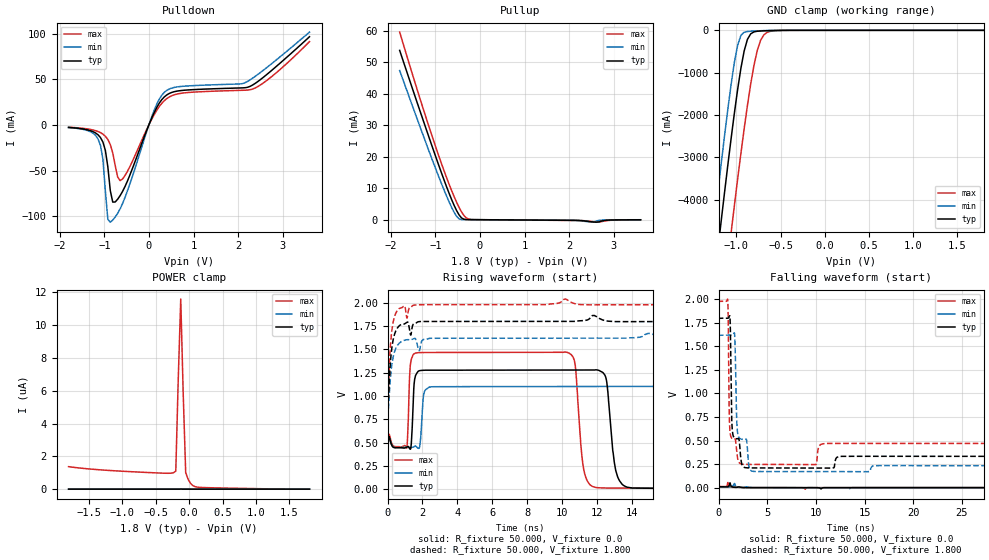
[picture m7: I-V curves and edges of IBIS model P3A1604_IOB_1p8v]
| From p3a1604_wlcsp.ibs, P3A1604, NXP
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[Model] P3A1604_IOB_1p8v
Model_type I/O
Polarity   Non-Inverting
Enable   Active-High
Vinl =  0.7915V
Vinh =  0.9305V
C_comp   5.4pF   5pF   5.9pF
[Model Spec]
Vinh   0.9305V   0.7875V   1.094V
Vinl   0.7915V   0.6765V   0.8965V
[Temperature Range]   27.000   -40.000   125
[Voltage Range]   1.800V   1.620V   1.980V
[Pullup Reference]   1.800V   1.620V   1.980V
[Pulldown Reference]   0.0V   0.0V   0.0V
[POWER Clamp Reference]   1.800V   1.620V   1.980V
[GND Clamp Reference]   0.0V   0.0V   0.0V
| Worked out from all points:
|   slope of the pulldown table from 0 to 0.27 V, typ, clamps not added: 10.2 ohm
|   slope of the pullup table from 0 to 0.27 V, typ, clamps not added: 10 kohm
|   GND clamp passes 1 mA (typ) near -0.48 V on its own axis
|   rising waveform, R_fixture 50.000, V_fixture 1.800: 20-80 % time 228ps typ, 242ps min, 212ps max; typ from 0.345 V to 1.8 V
|   falling waveform, R_fixture 50.000, V_fixture 1.800: 20-80 % time 162ps typ, 1.14ns min, 101ps max; typ from 1.8 V to 0.322 V
[Pulldown]
|Voltage   I(typ)   I(min)   I(max)
-1.8V     -2.845mA   -2.943mA   -2.588mA
-1.14V    -10.89mA   -15.42mA   -7.292mA
-1.03V    -18.9mA    -37.82mA   -10.16mA
-975mV    -28.05mA   -72.75mA   -12.51mA
-920mV    -45.98mA   -103.5mA   -16.01mA
-865mV    -72.04mA   -106.6mA   -21.57mA
-700mV    -81.45mA   -96.91mA   -57.13mA
-590mV    -72.88mA   -86.18mA   -59.25mA
70mV      8.156mA    9.743mA    6.781mA
345mV     30.59mA    35.56mA    26.48mA
2.27V     42.2mA     49.35mA    38.47mA
3.6V      96.53mA    101.6mA    91.18mA
[Pullup]
|Voltage   I(typ)   I(min)   I(max)
-1.8V     53.79mA    47.38mA    59.61mA
-1.185V   27.92mA    23.41mA    31.37mA
-910mV    16.73mA    13.15mA    19.72mA
-690mV    8.304mA    5.585mA    11.19mA
-580mV    4.559mA    2.361mA    7.344mA
-470mV    1.547mA    293.1uA    3.945mA
-415mV    584.4uA    60.57uA    2.504mA
-305mV    45.16uA    26.52uA    555.6uA
-140mV    13.98uA    12.12uA    10.95uA
2.5V      -675.5uA   -725.4uA   -572.1uA
2.665V    -692.6uA   -220.5uA   -748.4uA
3.6V      -27.43uA   -15.82uA   -42.87uA
[GND_clamp]
|Voltage   I(typ)   I(min)   I(max)
-1.8V     -16.4A     -15.08A    -18.65A
-1.282V   -6.516A    -5.156A    -8.809A
-1.245V   -5.834A    -4.473A    -8.124A
-1.171V   -4.49A     -3.137A    -6.77A
-1.06V    -2.563A    -1.283A    -4.789A
-1.023V   -1.963A    -760.5mA   -4.148A
-986mV    -1.401A    -351.8mA   -3.521A
-912mV    -488.2mA   -45.43mA   -2.328A
-838mV    -82.68mA   -20.71mA   -1.27A
-764mV    -21.98mA   -13.01mA   -479.2mA
-653mV    -9.053mA   -4.595mA   -49.07mA
1.8V      0A         0A         0A
[POWER_clamp]
|Voltage   I(typ)   I(min)   I(max)
-1.8V     3.151nA    587.7pA    1.372uA
-457mV    1.235nA    319.8pA    986.4nA
-272mV    1.169nA    343.5pA    974.1nA
-198mV    1.175nA    846.9pA    1.099uA
-161mV    1.276nA    342.9pA    6.758uA
-124mV    8.636nA    256.6pA    11.59uA
-87mV     2.849nA    235.6pA    5.78uA
-50mV     1.552nA    217.5pA    1.006uA
-13mV     752pA      172.3pA    592.5nA
24mV      396pA      107.1pA    343.1nA
172mV     160.3pA    62.42pA    105.9nA
1.8V      0A         0A         0A
[Ramp]
| variable   typ   min   max
dV/dt_r   5.356m/0.386p   4.190m/0.353p   7.055m/0.441p
dV/dt_f   0.887/0.164n   0.835/1.137n   0.916/99.242p
R_load = 50.000
[Rising Waveform]
R_fixture= 50.000
V_fixture= 0.0
V_fixture_min= 0.0
V_fixture_max= 0.0
|time   V(typ)   V(min)   V(max)
0s        800uV      500uV      1mV
1.1ns     451.3mV    448.7mV    445.6mV
1.52ns    1.131V     457.5mV    1.454V
2.36ns    1.277V     1.092V     1.467V
10.17ns   1.278V     1.101V     1.472V
11.31ns   1.278V     1.101V     158.7mV
12.63ns   1.049V     1.101V     12.45mV
13.45ns   52.66mV    1.101V     11.99mV
18.37ns   8.944mV    7.981mV    11.76mV
1us       8.927mV    6.983mV    11.76mV
[Rising Waveform]
R_fixture= 50.000
V_fixture= 1.800
V_fixture_min= 1.620
V_fixture_max= 1.980
|time   V(typ)   V(min)   V(max)
0s        345.1mV    251.6mV    474.6mV
10ps      652.2mV    575.8mV    741.4mV
30ps      883.9mV    803.4mV    975.9mV
180ps     1.406V     1.236V     1.587V
360ps     1.639V     1.452V     1.829V
640ps     1.749V     1.562V     1.935V
1.11ns    1.792V     1.605V     1.836V
1.33ns    1.654V     1.602V     1.953V
10.21ns   1.8V       1.62V      2.04V
1us       1.8V       1.62V      1.98V
[Falling Waveform]
R_fixture= 50.000
V_fixture= 0.0
V_fixture_min= 0.0
V_fixture_max= 0.0
|time   V(typ)   V(min)   V(max)
0s        9mV        7mV        13mV
790ps     8.926mV    6.983mV    10.62mV
940ps     7.883mV    7.018mV    54.6mV
1.16ns    51.65mV    6.805mV    10.34mV
1.31ns    13.04mV    7.297mV    4.778mV
1.62ns    3.058mV    44.05mV    6.756mV
1.72ns    2.274mV    19.85mV    7.888mV
8.89ns    657.7nV    3.69uV     -16.35mV
10.51ns   -14.26mV   1.302uV    614.8nV
1us       7.902nV    2.891nV    1.368uV
[Falling Waveform]
R_fixture= 50.000
V_fixture= 1.800
V_fixture_min= 1.620
V_fixture_max= 1.980
|time   V(typ)   V(min)   V(max)
0s        1.797V     1.618V     1.978V
930ps     1.799V     1.62V      1.993V
1.15ns    1.821V     1.62V      606.2mV
1.39ns    614.8mV    1.621V     521.9mV
1.64ns    525.8mV    1.62V      519.7mV
1.93ns    520.2mV    588.5mV    318.4mV
2.78ns    211.3mV    515.7mV    246.7mV
3.22ns    209.4mV    190.9mV    246.3mV
4.85ns    208.9mV    170.8mV    246mV
1us       322.1mV    229.2mV    453.1mV
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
